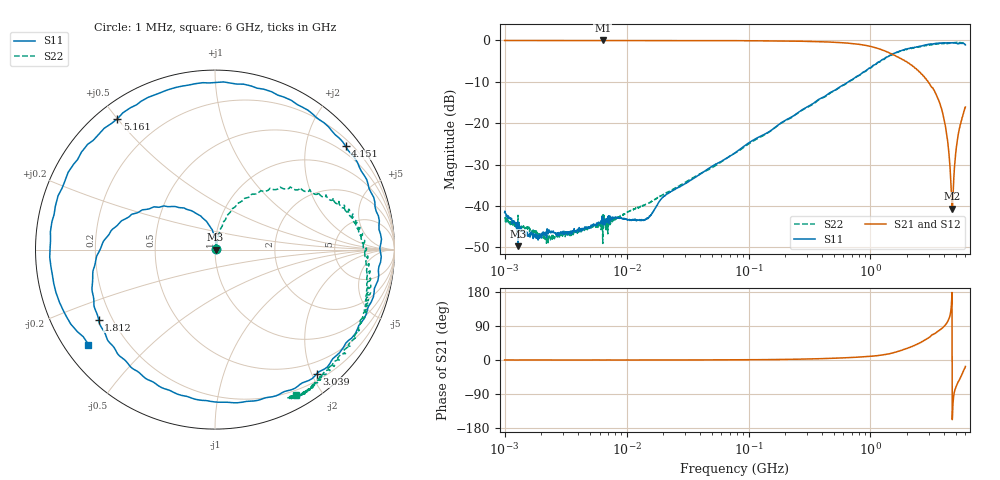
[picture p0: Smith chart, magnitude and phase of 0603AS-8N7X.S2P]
!s-Parameter Generated by FASTRON Sdn. Bhd.
!FASTRON P/N : 0603AS-8N7X
!Keysight Technologies: E5071C_MY46733604_B.14.02
!Date: Thu Nov 30 13:33:00 2023
!Version  :Rev01  Thu Nov 30 13:33:00 2023
!Data & Calibration Information:
!Freq  S11:SOLT2(ON)  S21:SOLT2(ON)  S12:SOLT2(ON)  S22:SOLT2(ON)
!PortZ  Port1:50+j0  Port2:50+j0
!When reading reference impedance value at option line is always used.
! Remarks : This data is being provided solely for informational purposes.
# Hz S dB R 50
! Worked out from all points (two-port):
!   1601 points, 1 MHz to 6 GHz, reference 50 ohm
!   highest |S21| = -0.03 dB at 6.378 MHz (marker M1); lowest = -40.7 dB at 4.685 GHz (marker M2)
!   |S21| within 3 dB of the highest: start of sweep to 1.422 GHz
!   lowest |S11| = -49.7 dB at 1.288 MHz (marker M3), VSWR 1.01, Z = 50.3 - j0.052 ohm
!   |S11| at or under -10 dB: start of sweep to 657.7 MHz
!   |S22| runs from -49.1 to -0.5 dB; largest |S21 - S12| = 0.0072
!   S11 on the Smith chart (normalised r, x): 1 MHz: 1.02, +0.00; 1.812 GHz: 0.15, -0.27; 3.039 GHz: 0.30, -2.08; 4.151 GHz: 0.34, +2.84; 5.161 GHz: 0.06, +0.50; 6 GHz: 0.07, -0.33
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1000000  -41.58 13.1  -0.04 0.1  -0.06 0.1  -42.97 17.2
1287650  -49.73 -9.1  -0.06 -0.0  -0.04 0.2  -42.28 3.8
2178434  -46.96 30.1  -0.05 0.0  -0.05 0.0  -48.00 34.3
4277066  -45.91 36.5  -0.05 0.0  -0.05 0.0  -46.07 39.1
6378092  -44.38 53.5  -0.03 0.0  -0.06 -0.1  -49.08 44.8
1.408869e7  -43.27 65.3  -0.05 0.0  -0.06 -0.0  -39.71 50.8
1.823719e7  -39.28 66.6  -0.05 0.0  -0.06 0.1  -37.87 61.5
7.757876e7  -27.18 84.8  -0.08 0.5  -0.09 0.5  -27.23 74.8
3.307917e8  -15.45 107.5  -0.27 2.9  -0.28 2.9  -15.60 72.3
8.87456e8  -7.57 145.5  -1.16 8.6  -1.16 8.5  -7.63 52.1
1.414819e9  -3.80 -179.1  -2.98 16.2  -2.99 16.1  -3.87 28.7
1.811747e9  -2.42 -149.0  -4.57 25.7  -4.59 25.6  -2.47 18.0
2.109383e9  -1.89 -125.9  -5.77 33.4  -5.80 33.3  -1.89 10.7
2.482341e9  -1.49 -96.0  -7.44 43.3  -7.45 43.3  -1.60 -0.4
3.039051e9  -0.97 -50.7  -10.41 60.0  -10.40 59.9  -1.17 -14.4
3.604213e9  -0.74 -5.9  -14.33 77.1  -14.31 76.9  -0.83 -26.6
4.150942e9  -0.65 38.4  -21.43 94.3  -21.43 94.0  -0.64 -44.5
4.517068e9  -0.59 70.2  -32.00 121.9  -32.01 121.6  -0.63 -51.8
4.684947e9  -0.62 84.7  -40.66 -157.4  -40.68 -157.6  -0.64 -54.3
5.160604e9  -0.83 126.9  -24.02 -62.4  -24.04 -62.5  -0.58 -58.5
5.580302e9  -0.71 170.3  -19.32 -40.5  -19.32 -40.6  -0.60 -62.9
6e9  -1.10 -143.1  -16.13 -17.2  -16.11 -17.3  -0.66 -60.8
